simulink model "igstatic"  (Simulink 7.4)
settings: Solver=ode45  StartTime=0.0  StopTime=20  MaxStep=1
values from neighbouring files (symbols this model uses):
  M = length(wmm)    [Actac.m]    (also in acttrcalc1.m = str2num(get(h,'string')); calc0.m = fix(tf/ti))
  Rr = input('Rotor resistance)[default = 2] =')    [Actac.m]    (also in im1phase.m = 0.3; im3d.m = eval(get(hRr,'String')); IMabc2.m = 0.02; imabcparam.m = 0.408)
  Rs = eval(get(hRs,'String'))    [im3d.m]    (also in IMabc2.m = 0.01; imabcparam.m = 0.531; IMabcrun0.m = 0.531; IMabcrun1.m = 0.531)
  Xm = input('Magnetizing reactance [default = 4.5] =')    [Actac.m]    (also in imdqsrkB.m = eval(get(hXm,'String')))
undefined symbols (not defined in the file or in its folder): Xlr, Xls
libraries: simulink_extras x1

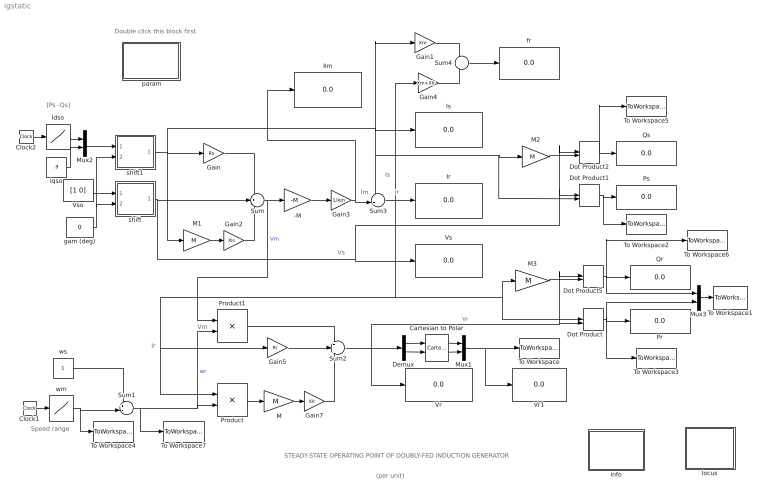
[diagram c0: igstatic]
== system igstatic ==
  note: Ir
  note: STEADY-STATE OPERATING POINT OF DOUBLY-FED INDUCTION GENERATOR
  note: Is
  note: Im
  note: [Ps -Qs]
  note: (per unit)
  note: Vs
  note: Double click this block first
  note: Vm
  note: Ir
  note: Speed range
  " param" : Subsystem
  -M : Gain  Gain=-M  Multiplication=Matrix(K*u)  ParameterDataType=sfix(16)  ParameterScaling=2^0  OutDataType=sfix(16)  OutScaling=2^0
  Cartesian to Polar : simulink_extras/Transformations/Cartesian to Polar  SystemSampleTime=-1
  Clock1 : Clock
  Clock2 : Clock
  Demux : Demux  Outputs=2
  Dot Product{,1..2,5} (4 alike) : DotProduct  OutDataType=fixdt(1, 16)  OutScaling=2^-10
  Gain : Gain  Gain=Rs  ParameterDataType=sfix(16)  ParameterScaling=2^0  OutDataType=sfix(16)  OutScaling=2^0
  Gain1 : Gain  Gain=Xm  ParameterDataType=sfix(16)  ParameterScaling=2^0  OutDataType=sfix(16)  OutScaling=2^0
  Gain2 : Gain  Gain=Xls  ParameterDataType=sfix(16)  ParameterScaling=2^0  OutDataType=sfix(16)  OutScaling=2^0
  Gain3 : Gain  Gain=1/Xm  ParameterDataType=sfix(16)  ParameterScaling=2^0  OutDataType=sfix(16)  OutScaling=2^0
  Gain4 : Gain  Gain=Xm+Xlr  ParameterDataType=sfix(16)  ParameterScaling=2^0  OutDataType=sfix(16)  OutScaling=2^0
  Gain5 : Gain  Gain=Rr  ParameterDataType=sfix(16)  ParameterScaling=2^0  OutDataType=sfix(16)  OutScaling=2^0
  Gain7 : Gain  Gain=Xlr  ParameterDataType=sfix(16)  ParameterScaling=2^0  OutDataType=sfix(16)  OutScaling=2^0
  IIm : Display
  Idso : Lookup  InputValues=[0 20 ]  Table=[-1 -1]  OutDataType=sfix(16)  OutScaling=2^0
  Iqso : Constant  Value=.9  OutDataType=sfix(16)  OutScaling=2^0
  Ir : Display
  Is : Display
  M{,1..3} (4 alike) : Gain  Gain=M  Multiplication=Matrix(K*u)  ParameterDataType=sfix(16)  ParameterScaling=2^0  OutDataType=sfix(16)  OutScaling=2^0
  Mux1 : Mux  Inputs=2
  Mux2 : Mux  Inputs=2
  Mux3 : Mux  Inputs=2
  Pr : Display
  Product : Product  OutDataType=sfix(16)  OutScaling=2^0
  Product1 : Product  OutDataType=sfix(16)  OutScaling=2^0
  Ps : Display
  Qr : Display
  Qs : Display
  Sum : Sum  Inputs=-+-  OutDataType=sfix(16)  OutScaling=2^0
  Sum1 : Sum  Inputs=+-|  OutDataType=sfix(16)  OutScaling=2^0
  Sum2 : Sum  Inputs=+++  OutDataType=sfix(16)  OutScaling=2^0
  Sum3 : Sum  Inputs=-+|  OutDataType=sfix(16)  OutScaling=2^0
  Sum4 : Sum  OutDataType=sfix(16)  OutScaling=2^0
  To Workspace : ToWorkspace  VariableName=V  SampleTime=-1  SaveFormat=Array
  To Workspace1 : ToWorkspace  VariableName=PQ  SampleTime=-1  SaveFormat=Array
  To Workspace2 : ToWorkspace  VariableName=Ps  SampleTime=-1  SaveFormat=Array
  To Workspace3 : ToWorkspace  VariableName=Pr  SampleTime=-1  SaveFormat=Array
  To Workspace4 : ToWorkspace  VariableName=wm  SampleTime=-1  SaveFormat=Array
  To Workspace5 : ToWorkspace  VariableName=Qs  SampleTime=-1  SaveFormat=Array
  To Workspace6 : ToWorkspace  VariableName=Qr  SampleTime=-1  SaveFormat=Array
  To Workspace7 : ToWorkspace  VariableName=wr  SampleTime=-1  SaveFormat=Array
  Vr : Display
  Vr1 : Display
  Vs : Display
  Vso : Constant  Value=[1 0]  OutDataType=sfix(16)  OutScaling=2^0
  fr : Display
  gam (deg) : Constant  Value=0  OutDataType=sfix(16)  OutScaling=2^0
  info : Subsystem
  locus : Subsystem
  shift : Subsystem
  shift1 : Subsystem
  wm : Lookup  InputValues=[0 20 ]  Table=[.7 1.3]  OutDataType=sfix(16)  OutScaling=2^0
  ws : Constant  OutDataType=sfix(16)  OutScaling=2^0
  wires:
  Gain/1 -> Sum/1
  M1/1 -> Gain2/1
  Gain2/1 -> Sum/3
  -M/1 -> Gain3/1
  Gain5/1 -> Sum2/2
  Sum1/1 -> Product/2, Product1/2, To Workspace7/1  "wr"
  M/1 -> Gain7/1
  Product/1 -> M/1
  Gain7/1 -> Sum2/3
  Product1/1 -> Sum2/1
  Sum2/1 -> Dot Product5/1, Dot Product/2, Vr/1, Demux/1  "Vr"
  Sum3/1 -> Product/1, Gain5/1, M3/1, Dot Product/1, Ir/1, Gain4/1
  Vso/1 -> shift/1(vso)
  shift/1(vs) -> Sum/2, Vs/1, Dot Product2/1, Dot Product1/1
  gam (deg)/1 -> shift/2(gama), shift1/2(gama)
  shift1/1(is) -> Gain/1, M1/1, Sum3/1, M2/1, Dot Product1/2, Is/1, Gain1/1
  Dot Product/1 -> Pr/1, Mux3/2, To Workspace3/1
  M3/1 -> Dot Product5/2
  Dot Product1/1 -> Ps/1, To Workspace2/1
  Dot Product2/1 -> Qs/1, To Workspace5/1
  M2/1 -> Dot Product2/2
  Demux/1 -> Cartesian to Polar/1
  Demux/2 -> Cartesian to Polar/2
  Cartesian to Polar/1 -> Mux1/1
  Cartesian to Polar/2 -> Mux1/2
  Sum/1 -> -M/1, Product1/1  "Vm"
  Mux1/1 -> Vr1/1, To Workspace/1
  Clock1/1 -> wm/1
  wm/1 -> Sum1/2, To Workspace4/1
  ws/1 -> Sum1/1
  Mux2/1 -> shift1/1(iso)
  Clock2/1 -> Idso/1
  Idso/1 -> Mux2/1
  Iqso/1 -> Mux2/2
  Dot Product5/1 -> Qr/1, Mux3/1, To Workspace6/1
  Mux3/1 -> To Workspace1/1
  Gain1/1 -> Sum4/1
  Gain4/1 -> Sum4/2
  Sum4/1 -> fr/1
  Gain3/1 -> Sum3/2, IIm/1

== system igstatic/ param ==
  note: Double click the block to enter the parameters

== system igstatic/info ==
  note: Phasor equations of the induction machine in steady state obtained from the standard per-phase equivalent circuit. (Per-unit formulation)
  note: Vs = (Rs+jXls) Is + Vm Vr = sVm + (Rr+jsXlr) Ir Im = Vm / (jXm) Is + Ir = Im s = wr = ws - wm
  note: INPUTS: Vs and Is ; wm OUTPUT: Vr

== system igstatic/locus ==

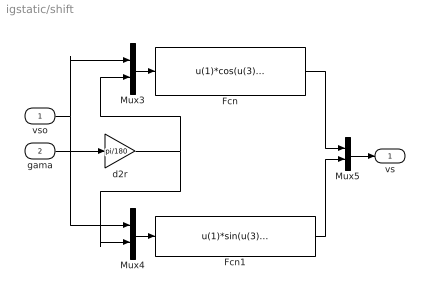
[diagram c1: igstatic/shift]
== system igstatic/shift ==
  vso : Inport  OutDataType=sfix(16)  OutScaling=2^0
  gama : Inport  Port=2  OutDataType=sfix(16)  OutScaling=2^0
  Fcn : Fcn  Expr=u(1)*cos(u(3))-u(2)*sin(u(3))
  Fcn1 : Fcn  Expr=u(1)*sin(u(3))+u(2)*cos(u(3))
  Mux3 : Mux  Inputs=2
  Mux4 : Mux  Inputs=2
  Mux5 : Mux  Inputs=2
  d2r : Gain  Gain=pi/180  Multiplication=Matrix(K*u)  ParameterDataType=sfix(16)  ParameterScaling=2^0  OutDataType=sfix(16)  OutScaling=2^0
  vs : Outport
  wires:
  Mux3/1 -> Fcn/1
  Mux4/1 -> Fcn1/1
  vso/1 -> Mux3/1, Mux4/1
  gama/1 -> d2r/1
  Fcn1/1 -> Mux5/2
  Fcn/1 -> Mux5/1
  Mux5/1 -> vs/1
  d2r/1 -> Mux3/2, Mux4/2

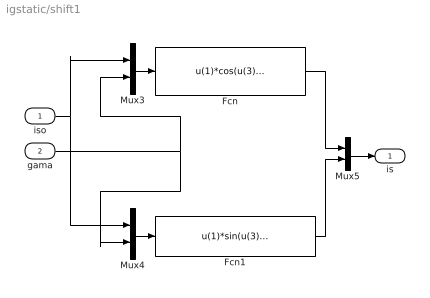
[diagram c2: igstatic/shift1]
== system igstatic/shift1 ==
  iso : Inport  OutDataType=sfix(16)  OutScaling=2^0
  gama : Inport  Port=2  OutDataType=sfix(16)  OutScaling=2^0
  Fcn : Fcn  Expr=u(1)*cos(u(3))-u(2)*sin(u(3))
  Fcn1 : Fcn  Expr=u(1)*sin(u(3))+u(2)*cos(u(3))
  Mux3 : Mux  Inputs=2
  Mux4 : Mux  Inputs=2
  Mux5 : Mux  Inputs=2
  is : Outport
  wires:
  Mux5/1 -> is/1
  Fcn/1 -> Mux5/1
  Fcn1/1 -> Mux5/2
  gama/1 -> Mux4/2, Mux3/2
  iso/1 -> Mux4/1, Mux3/1
  Mux4/1 -> Fcn1/1
  Mux3/1 -> Fcn/1
